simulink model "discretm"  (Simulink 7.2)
settings: Solver=FixedStepDiscrete  StartTime=0.0  StopTime=15  FixedStep=Ts  RelTol=1e-3
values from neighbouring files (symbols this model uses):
  a = -1.1    [derive_init.m]    (also in discretm_init.m)
  b = .2    (= 0.2)    [derive_init.m]    (also in discretm_init.m)
  K = .15    (= 0.15)    [derive_init.m]    (also in discretm_init.m)
  Ts = .1    (= 0.1)    [derive_init.m]    (also in discretm_init.m)
undefined symbols (not defined in the file or in its folder): DiscIntNeverNeededParam

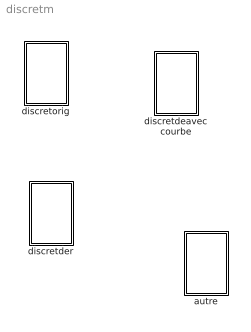
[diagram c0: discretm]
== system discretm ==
  autre : Subsystem
  discretdeavec courbe : Subsystem
  discretder : Subsystem
  discretorig : Subsystem

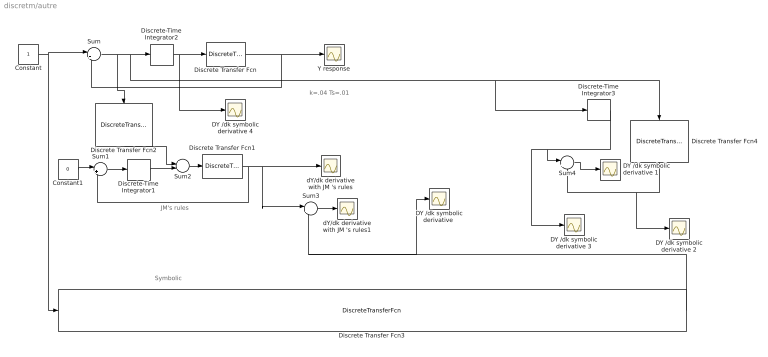
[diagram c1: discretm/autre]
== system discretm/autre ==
  note: k=.04 Ts=.01
  note: Symbolic
  note: JM's rules
  Constant : Constant  OutDataType=sfix(16)  OutScaling=2^0
  Constant1 : Constant  Value=0  OutDataType=sfix(16)  OutScaling=2^0
  DY /dk symbolic derivative {,1..4} (5 alike) : Scope
  Discrete Transfer Fcn : DiscreteTransferFcn  Numerator=[1 ]  Denominator="[1   b]"  SampleTime=-1
  Discrete Transfer Fcn1 : DiscreteTransferFcn  Numerator=[1 ]  Denominator="[1  b]"  SampleTime=-1
  Discrete Transfer Fcn2 : DiscreteTransferFcn  Orientation=down  Numerator=Ts  Denominator="[1  -1]"  SampleTime=-1
  Discrete Transfer Fcn3 : DiscreteTransferFcn  Numerator="[ Ts  (Ts + Ts * (a - 1))   (Ts * (a - 1) + Ts * (K * Ts - a + b) - K * Ts ^ 2)   (Ts * (K * Ts - a + b) + Ts * (K * Ts - b) - 2 * K * Ts ^ 2)   Ts * (K * Ts - b) - K * Ts ^ 2]"  Denominator="[1   (2 * a - 2)    (2 * K * Ts - 2 * a + 2 * b + (a - 1) ^ 2)    (2 * K * Ts - 2 * b + 2 * (K * Ts - a + b) * (a - 1))    (2 * (K * Ts - b) * (a - 1) + (K * Ts - a + b) ^ 2)    2 * (K * Ts - b) * (K * Ts - a + b)   (K * Ts - b) ^ 2]"  SampleTime=-1
  Discrete Transfer Fcn4 : DiscreteTransferFcn  Orientation=down  Numerator=Ts  Denominator="[1  -1]"  SampleTime=-1
  Discrete-Time Integrator1 : DiscreteIntegrator  gainval=K  SampleTime=-1  OutDataType=sfix(16)  OutScaling=2^0  ICPrevOutput=DiscIntNeverNeededParam  ICPrevScaledInput=DiscIntNeverNeededParam
  Discrete-Time Integrator2 : DiscreteIntegrator  gainval=K  SampleTime=-1  OutDataType=sfix(16)  OutScaling=2^0  ICPrevOutput=DiscIntNeverNeededParam  ICPrevScaledInput=DiscIntNeverNeededParam
  Discrete-Time Integrator3 : DiscreteIntegrator  gainval=1  SampleTime=Ts  OutDataType=sfix(16)  OutScaling=2^0  ICPrevOutput=DiscIntNeverNeededParam  ICPrevScaledInput=DiscIntNeverNeededParam
  Sum{,1,3..4} (4 alike) : Sum  Inputs=|+-  OutDataType=sfix(16)  OutScaling=2^0
  Sum2 : Sum  OutDataType=sfix(16)  OutScaling=2^0
  Y response : Scope
  dY/dk derivative with JM 's rules : Scope
  dY/dk derivative with JM 's rules1 : Scope
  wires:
  Discrete Transfer Fcn/1 -> Sum/2, Y response/1
  Sum/1 -> Discrete-Time Integrator2/1, Discrete Transfer Fcn4/1, Discrete-Time Integrator3/1, Discrete Transfer Fcn2/1
  Constant/1 -> Sum/1, Discrete Transfer Fcn3/1
  Discrete Transfer Fcn1/1 -> Sum1/2, dY/dk derivative with JM 's rules/1, Sum3/1
  Sum1/1 -> Discrete-Time Integrator1/1
  Constant1/1 -> Sum1/1
  Discrete-Time Integrator2/1 -> Discrete Transfer Fcn/1, DY /dk symbolic derivative 4/1
  Sum2/1 -> Discrete Transfer Fcn1/1
  Discrete-Time Integrator1/1 -> Sum2/2
  Discrete Transfer Fcn2/1 -> Sum2/1
  Discrete Transfer Fcn3/1 -> "DY /dk symbolic derivative "/1, Sum3/2
  Sum3/1 -> dY/dk derivative with JM 's rules1/1
  Discrete-Time Integrator3/1 -> Sum4/1, DY /dk symbolic derivative 3/1
  Discrete Transfer Fcn4/1 -> Sum4/2, DY /dk symbolic derivative 2/1
  Sum4/1 -> DY /dk symbolic derivative 1/1

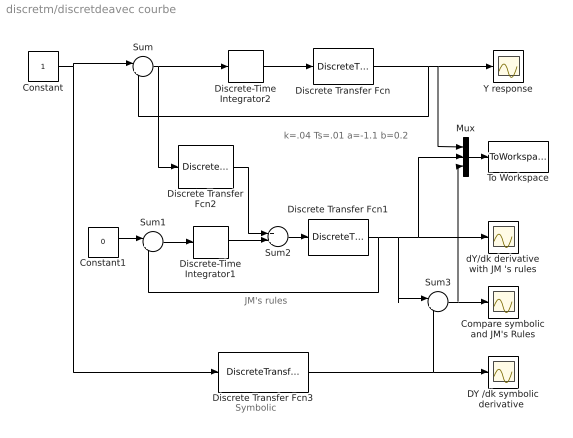
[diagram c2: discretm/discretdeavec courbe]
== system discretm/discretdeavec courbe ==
  note: k=.04 Ts=.01 a=-1.1 b=0.2
  note: JM's rules
  note: Symbolic
  Compare symbolic and JM's Rules : Scope
  Constant : Constant  OutDataType=sfix(16)  OutScaling=2^0
  Constant1 : Constant  Value=0  OutDataType=sfix(16)  OutScaling=2^0
  "DY /dk symbolic derivative " : Scope
  Discrete Transfer Fcn : DiscreteTransferFcn  Numerator=[1 +1]  Denominator="[1 a  b]"  SampleTime=-1
  Discrete Transfer Fcn1 : DiscreteTransferFcn  Numerator=[1 1]  Denominator=[1 a b]  SampleTime=-1
  Discrete Transfer Fcn2 : DiscreteTransferFcn  Numerator=Ts  Denominator="[1  -1]"  SampleTime=-1
  Discrete Transfer Fcn3 : DiscreteTransferFcn  Numerator="[ Ts  (Ts + Ts * (a - 1))   (Ts * (a - 1) + Ts * (K * Ts - a + b) - K * Ts ^ 2)   (Ts * (K * Ts - a + b) + Ts * (K * Ts - b) - 2 * K * Ts ^ 2)   Ts * (K * Ts - b) - K * Ts ^ 2]"  Denominator="[1   (2 * a - 2)    (2 * K * Ts - 2 * a + 2 * b + (a - 1) ^ 2)    (2 * K * Ts - 2 * b + 2 * (K * Ts - a + b) * (a - 1))    (2 * (K * Ts - b) * (a - 1) + (K * Ts - a + b) ^ 2)    2 * (K * Ts - b) * (K * Ts - a + b)   (K * Ts - b) ^ 2]"  SampleTime=-1
  Discrete-Time Integrator1 : DiscreteIntegrator  gainval=K  SampleTime=-1  OutDataType=sfix(16)  OutScaling=2^0  ICPrevOutput=DiscIntNeverNeededParam  ICPrevScaledInput=DiscIntNeverNeededParam
  Discrete-Time Integrator2 : DiscreteIntegrator  gainval=K  SampleTime=-1  OutDataType=sfix(16)  OutScaling=2^0  ICPrevOutput=DiscIntNeverNeededParam  ICPrevScaledInput=DiscIntNeverNeededParam
  Mux : Mux  Inputs=3
  Sum : Sum  Inputs=|+-  OutDataType=sfix(16)  OutScaling=2^0
  Sum1 : Sum  Inputs=|+-  OutDataType=sfix(16)  OutScaling=2^0
  Sum2 : Sum  OutDataType=sfix(16)  OutScaling=2^0
  Sum3 : Sum  Inputs=|+-  OutDataType=sfix(16)  OutScaling=2^0
  To Workspace : ToWorkspace  VariableName=simout  SampleTime=-1  SaveFormat=Structure With Time
  Y response : Scope
  dY/dk derivative with JM 's rules : Scope
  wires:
  Sum3/1 -> Compare symbolic and JM's Rules/1, Mux/3
  Discrete Transfer Fcn3/1 -> Sum3/2, "DY /dk symbolic derivative "/1
  Discrete Transfer Fcn2/1 -> Sum2/1
  Discrete-Time Integrator1/1 -> Sum2/2
  Sum2/1 -> Discrete Transfer Fcn1/1
  Discrete-Time Integrator2/1 -> Discrete Transfer Fcn/1
  Constant1/1 -> Sum1/1
  Sum1/1 -> Discrete-Time Integrator1/1
  Discrete Transfer Fcn1/1 -> Sum3/1, Mux/2, dY/dk derivative with JM 's rules/1, Sum1/2
  Constant/1 -> Discrete Transfer Fcn3/1, Sum/1
  Sum/1 -> Discrete Transfer Fcn2/1, Discrete-Time Integrator2/1
  Discrete Transfer Fcn/1 -> Sum/2, Y response/1, Mux/1
  Mux/1 -> To Workspace/1

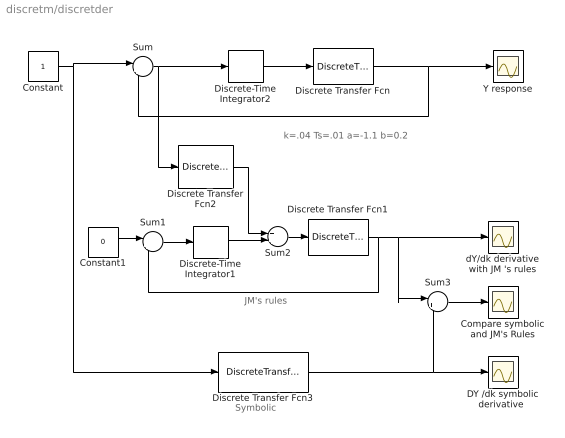
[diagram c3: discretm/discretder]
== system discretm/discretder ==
  note: Symbolic
  note: JM's rules
  note: k=.04 Ts=.01 a=-1.1 b=0.2
  Compare symbolic and JM's Rules : Scope
  Constant : Constant  OutDataType=sfix(16)  OutScaling=2^0
  Constant1 : Constant  Value=0  OutDataType=sfix(16)  OutScaling=2^0
  "DY /dk symbolic derivative " : Scope
  Discrete Transfer Fcn : DiscreteTransferFcn  Numerator=[1 +1]  Denominator="[1 a  b]"  SampleTime=-1
  Discrete Transfer Fcn1 : DiscreteTransferFcn  Numerator=[1 1]  Denominator=[1 a b]  SampleTime=-1
  Discrete Transfer Fcn2 : DiscreteTransferFcn  Numerator=Ts  Denominator="[1  -1]"  SampleTime=-1
  Discrete Transfer Fcn3 : DiscreteTransferFcn  Numerator="[ Ts  (Ts + Ts * (a - 1))   (Ts * (a - 1) + Ts * (K * Ts - a + b) - K * Ts ^ 2)   (Ts * (K * Ts - a + b) + Ts * (K * Ts - b) - 2 * K * Ts ^ 2)   Ts * (K * Ts - b) - K * Ts ^ 2]"  Denominator="[1   (2 * a - 2)    (2 * K * Ts - 2 * a + 2 * b + (a - 1) ^ 2)    (2 * K * Ts - 2 * b + 2 * (K * Ts - a + b) * (a - 1))    (2 * (K * Ts - b) * (a - 1) + (K * Ts - a + b) ^ 2)    2 * (K * Ts - b) * (K * Ts - a + b)   (K * Ts - b) ^ 2]"  SampleTime=-1
  Discrete-Time Integrator1 : DiscreteIntegrator  gainval=K  SampleTime=-1  OutDataType=sfix(16)  OutScaling=2^0  ICPrevOutput=DiscIntNeverNeededParam  ICPrevScaledInput=DiscIntNeverNeededParam
  Discrete-Time Integrator2 : DiscreteIntegrator  gainval=K  SampleTime=-1  OutDataType=sfix(16)  OutScaling=2^0  ICPrevOutput=DiscIntNeverNeededParam  ICPrevScaledInput=DiscIntNeverNeededParam
  Sum : Sum  Inputs=|+-  OutDataType=sfix(16)  OutScaling=2^0
  Sum1 : Sum  Inputs=|+-  OutDataType=sfix(16)  OutScaling=2^0
  Sum2 : Sum  OutDataType=sfix(16)  OutScaling=2^0
  Sum3 : Sum  Inputs=|+-  OutDataType=sfix(16)  OutScaling=2^0
  Y response : Scope
  dY/dk derivative with JM 's rules : Scope
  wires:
  Discrete Transfer Fcn/1 -> Sum/2, Y response/1
  Sum/1 -> Discrete-Time Integrator2/1, Discrete Transfer Fcn2/1
  Constant/1 -> Sum/1, Discrete Transfer Fcn3/1
  Discrete Transfer Fcn1/1 -> Sum1/2, dY/dk derivative with JM 's rules/1, Sum3/1
  Sum1/1 -> Discrete-Time Integrator1/1
  Constant1/1 -> Sum1/1
  Discrete-Time Integrator2/1 -> Discrete Transfer Fcn/1
  Sum2/1 -> Discrete Transfer Fcn1/1
  Discrete-Time Integrator1/1 -> Sum2/2
  Discrete Transfer Fcn2/1 -> Sum2/1
  Discrete Transfer Fcn3/1 -> "DY /dk symbolic derivative "/1, Sum3/2
  Sum3/1 -> Compare symbolic and JM's Rules/1

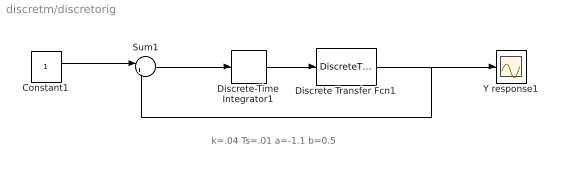
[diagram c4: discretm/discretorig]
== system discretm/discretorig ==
  note: k=.04 Ts=.01 a=-1.1 b=0.5
  Constant1 : Constant  OutDataType=sfix(16)  OutScaling=2^0
  Discrete Transfer Fcn1 : DiscreteTransferFcn  Numerator=[1 +1]  Denominator="[1 a  b]"  SampleTime=-1
  Discrete-Time Integrator1 : DiscreteIntegrator  gainval=K  SampleTime=-1  OutDataType=sfix(16)  OutScaling=2^0  ICPrevOutput=DiscIntNeverNeededParam  ICPrevScaledInput=DiscIntNeverNeededParam
  Sum1 : Sum  Inputs=|+-  OutDataType=sfix(16)  OutScaling=2^0
  Y response1 : Scope
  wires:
  Discrete Transfer Fcn1/1 -> Sum1/2, Y response1/1
  Sum1/1 -> Discrete-Time Integrator1/1
  Constant1/1 -> Sum1/1
  Discrete-Time Integrator1/1 -> Discrete Transfer Fcn1/1
